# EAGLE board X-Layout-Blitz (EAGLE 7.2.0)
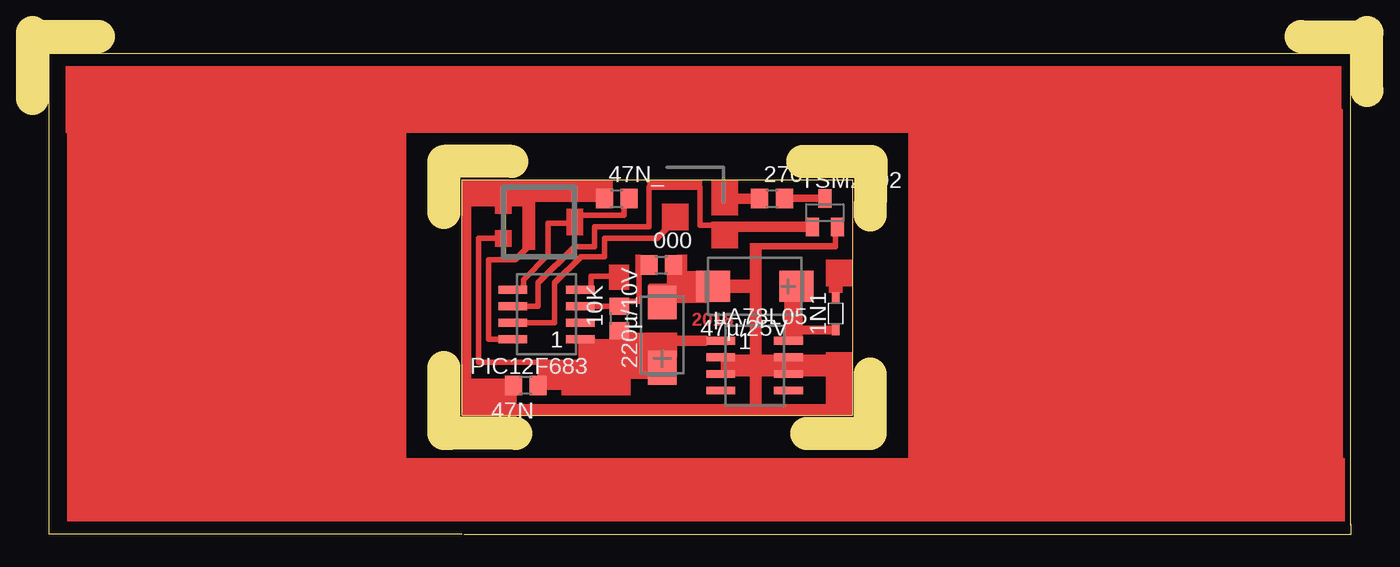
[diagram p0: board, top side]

Size 102.55 x 38.54 mm. Coordinates in mm from the lower left corner, seen from the top.
Outline: 37.15,7.75 32.07,7.75
Outline: 31.62,7.75 31.62,12.83
Outline: 59.5,7.75 64.39,7.75 64.39,12.32
Outline: 36.83,28.64 31.62,28.64 31.62,24.7
Outline: 64.39,24.51 64.45,28.58
Outline: 59.18,28.64 64.45,28.64
Outline: 101.28,0.7 101.28,36.96 1.27,36.96 1.27,0 33.02,0
Outline: 5.08,38.23 0,38.23
Outline: 0,33.46 0,38.23
Outline: 0,38.23 0,38.55
Outline: 102.55,34.1 102.55,38.55
Outline: 97.47,38.23 102.24,38.23
Outline: 33.15,0 101.35,0 101.35,0.76
Outline: 33.02,9.14 62.99,9.14 62.99,27.24 33.02,27.24 33.02,9.14
Copper layers (1*16): Top 0.035mm / dielectric 1.5mm / Bottom 0.035mm
Design rules "default": minimum track width 10mil, minimum drill 24mil, track to track 8mil, track to pad 8mil, pad to pad 8mil, via to via 8mil, smd to smd 8mil, copper to edge 40mil, drill to drill 8mil, minimum pad ring 10mil, minimum via ring 8mil, stop-mask expansion 4mil, vias tented up to drill 0mil, thermal gap 10mil

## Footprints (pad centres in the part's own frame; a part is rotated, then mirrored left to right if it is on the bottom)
R0805 = smd 1.3 x 1.5: 1 -0.95,0; 2 0.95,0
SOD323R_INFINEON = smd 0.8 x 0.6: A 1.25,0; C -1.25,0
CT7343 = smd 2.6 x 2.4: + -3.2,0; - 3.2,0
CT6032 = smd 2.6 x 2.2: + -2.5,0; - 2.5,0
SOP08 = smd 0.6 x 2.2: 1 -1.905,-2.6; 2 -0.635,-2.6; 3 0.635,-2.6; 4 1.905,-2.6; 5 1.905,2.6; 6 0.635,2.6; 7 -0.635,2.6; 8 -1.905,2.6
SOT23 = smd 1 x 1.4: 1 -0.95,-1.1; 2 0.95,-1.1; 3 0,1.1

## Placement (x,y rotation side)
000  [R0805]  48.32,20.7 0 top
1N1  [SOD323R_INFINEON]  61.72,16.95 90 top
10K  [R0805]  45.09,16.57 90 top
47N  [R0805]  37.91,11.43 180 top
47N_  [R0805]  44.89,25.78 0 top
47µ/25V  [CT7343]  55.5,19.05 180 top
220µ/10V  [CT6032]  48.39,15.3 90 top
270  [R0805]  56.83,25.78 0 top
PIC12F683  [SOP08]  39.5,16.89 90 top
TSM2302  [SOT23]  60.9,24.7 0 top
µA78L05  [SOP08]  55.5,12.95 270 top

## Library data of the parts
000 10K 47N 47N_ 47µ/25V 220µ/10V 270 PIC12F683 TSM2302 µA78L05 = smd-ipc
1N1 = diode

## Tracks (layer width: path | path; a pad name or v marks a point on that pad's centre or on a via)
S$1
  Top 0.406: 43.05,14.35 44.45,14.35 | 43.05,14.35 43.05,14.99 | 42.16,14.99 42.16,14.35 | 42.16,14.35 42.16,11.3 | 42.16,11.3 38.99,11.3 | 38.99,11.3 38.86,11.43 | 38.99,11.3 38.99,13.21 | 38.99,13.21 34.29,13.21 34.29,22.73 36.2,22.73 | 43.05,14.35 42.16,14.35 | 38.99,13.21 42.29,13.21 | 42.16,11.3 45.59,11.3 45.59,12.83
S$2
  Top 0.406: 42.93,17.53 44.83,17.53
S$3
  Top 0.406: 61.72,18.29 61.72,20.07
S$4
  Top 0.406: 59.82,23.62 53.34,23.62
S$5
  Top 0.406: 58.67,13.59 61.59,13.59 61.59,12.32 55.5,12.32 | 55.5,12.32 53.09,12.32 53.09,13.59 57.79,13.59 | 55.5,12.32 55.5,9.78 | 55.5,9.78 36.58,9.78 | 36.58,9.78 36.58,11.68 | 36.58,9.78 33.53,9.78 33.53,25.4 36.2,25.4 | 55.5,9.78 61.34,9.78
S$6
  Top 0.406: 58.67,18.29 58.67,15.62 | 58.67,15.62 58.67,14.86 | 61.72,15.62 58.67,15.62
S$7
  Top 0.406: 52.32,14.86 48.39,14.86 48.39,13.72 | 48.39,13.72 48.39,12.06 | 48.39,13.72 44.45,13.72
S$8
  Top 0.406: 61.72,23.5 61.72,22.1 55.5,22.1 55.5,19.05 47.5,19.05 48.39,17.02
S$9
  Top 0.406: 37.72,18.8 37.72,19.56 39.62,21.46 39.62,23.88 41.66,23.88
S$11
  Top 0.406: 35.94,14.99 35.05,14.99 35.05,21.08 37.08,21.08 37.59,21.59 37.85,21.84 | 37.85,21.84 37.85,25.4 | 37.85,25.4 36.45,25.4 | 37.85,25.4 37.85,26.29 43.56,26.29 | 37.85,21.84 38.1,22.1
S$12
  Top 0.406: 49.28,20.83 49.28,18.8
S$13
  Top 0.406: 47.24,21.08 47.62,21.08
S$14
  Top 0.406: 46.61,21.08 46.61,17.91 45.34,17.91
S$15
  Top 0.406: 52.58,23.11 52.7,23.24
S$16
  Top 0.406: 45.47,25.4 45.47,24.51 41.78,24.51
S$17
  Top 0.406: 37.85,17.53 38.86,17.53 38.86,19.3 41.66,22.1 43.18,22.1 43.18,23.62 47.37,23.62 47.37,24.89 47.37,25.02 47.37,26.67 51.31,26.67 51.31,23.75 52.58,23.75
S$18
  Top 0.406: 57.79,25.91 60.71,25.91
S$19
  Top 0.406: 55.88,25.78 53.34,25.78
S$20
  Top 0.406: 37.72,16.26 40.13,16.26 40.13,19.3 42.16,21.34 43.94,21.34 43.94,22.73 47.88,22.73
S$21
  Top 0.406: 48.01,22.73 49.66,24.38
S$22
  Top 0.406: 42.93,18.8 42.93,19.81 44.7,19.81
(copper drawn outside any net)
  shapes: Top area x53

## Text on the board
Top: 2018
tDocu: LED-Anode | 5K | Data | Clock | Vpp | +9V bis +22V | Masse | +5V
